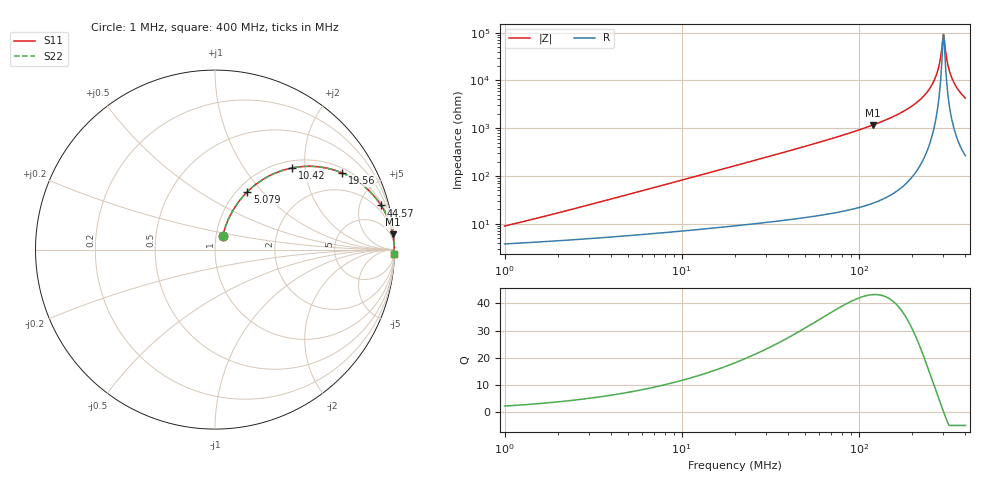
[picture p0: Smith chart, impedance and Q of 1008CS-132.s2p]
# MHz S MA R 50
!Freq  MagS11  AngS11  MagS21  AngS21  MagS12  AngS12  MagS22  AngS22
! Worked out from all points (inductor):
!   801 points, 1 MHz to 400 MHz, reference 50 ohm
!   read as one part in series: L = 1.3 uH near 1.532 MHz
!   highest Q = 43.2 at 119.8 MHz (marker M1), where L = 1.54 uH
!   self-resonance near 300.9 MHz
!   S11 on the Smith chart (normalised r, x): 1 MHz: 1.08, +0.16; 5.079 MHz: 1.11, +0.83; 10.42 MHz: 1.14, +1.71; 19.56 MHz: 1.18, +3.21; 44.57 MHz: 1.26, +7.44; 400 MHz: 6, -85
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1  0.08652 60.6  0.9604 -4.5  0.9604 -4.5  0.08652 60.6
2.728004  0.2128 65.9  0.9335 -12.0  0.9335 -12.0  0.2128 65.9
5.079357  0.3689 60.8  0.8808 -21.4  0.8808 -21.4  0.3689 60.8
7.38648  0.4963 54.4  0.8175 -29.6  0.8175 -29.6  0.4963 54.4
10.42452  0.6248 46.7  0.7303 -38.5  0.7303 -38.5  0.6248 46.7
19.55565  0.8284 31.0  0.5156 -55.8  0.5156 -55.8  0.8284 31.0
20  0.8341 30.4  0.5075 -56.4  0.5075 -56.4  0.8341 30.4
44.57132  0.9576 14.9  0.2571 -73.1  0.2571 -73.1  0.9576 14.9
54.56009  0.9711 12.2  0.2107 -76.1  0.2107 -76.1  0.9711 12.2
119.7831  0.9944 4.9  0.08553 -83.8  0.08553 -83.8  0.9944 4.9
147.7296  0.9965 3.6  0.06269 -85.0  0.06269 -85.0  0.9965 3.6
200.8275  0.9983 1.9  0.03378 -86.2  0.03378 -86.2  0.9983 1.9
245.8344  0.9988 0.9  0.0166 -85.5  0.0166 -85.5  0.9988 0.9
275.0624  0.9989 0.4  0.007419 -81.5  0.007419 -81.5  0.9989 0.4
283.4272  0.9989 0.3  0.005018 -77.6  0.005018 -77.6  0.9989 0.3
294.2418  0.9989 0.1  0.002151 -59.9  0.002151 -59.9  0.9989 0.1
300.9277  0.9989 0.0  0.001091 -2.0  0.001091 -2.0  0.9989 0.0
307.7655  0.9989 -0.1  0.002102 58.1  0.002102 58.1  0.9989 -0.1
321.9106  0.9988 -0.3  0.005558 77.8  0.005558 77.8  0.9988 -0.3
336.7059  0.9988 -0.5  0.009179 82.0  0.009179 82.0  0.9988 -0.5
362.8913  0.9986 -0.9  0.0153 84.3  0.0153 84.3  0.9986 -0.9
400  0.9983 -1.3  0.02341 85.1  0.02341 85.1  0.9983 -1.3
